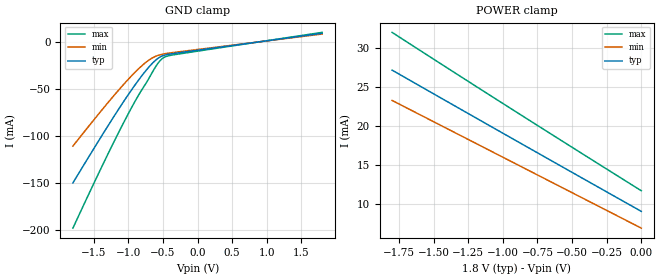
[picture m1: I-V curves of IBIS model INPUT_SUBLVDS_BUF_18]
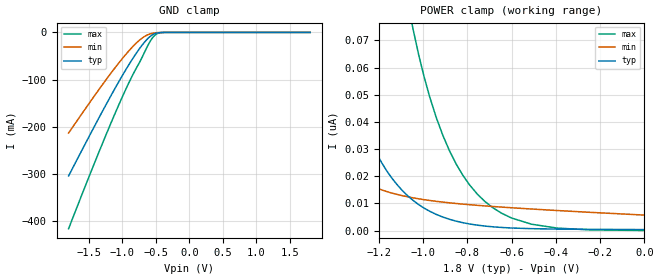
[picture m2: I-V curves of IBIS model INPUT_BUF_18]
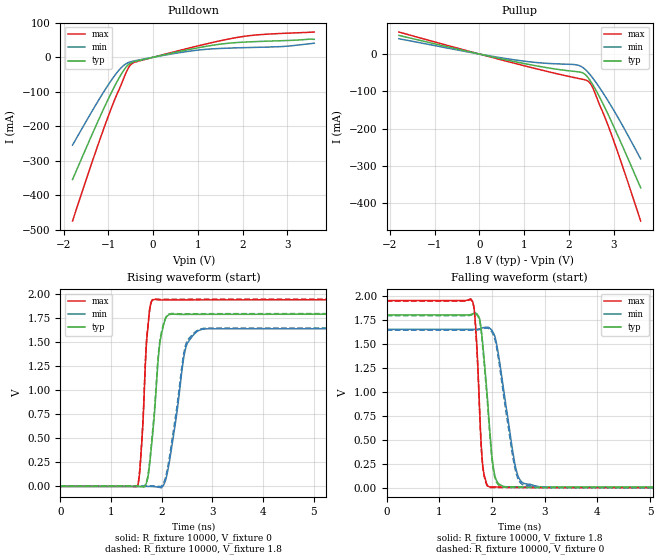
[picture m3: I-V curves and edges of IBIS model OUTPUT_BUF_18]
| TEXAS INSTRUMENTS INCORPORATED
| DLP Products
| IBIS Model of D1019WT7SV
| DLP4710 DMD
| This device can be powered at the following Vccs:
|  1.8 volt Vcc
| This file provides unique models under the [Model Selector] for each Vcc.
| For operation at a specific Vcc, select the appropriate model after each
| [Model Selector] keyword.
[IBIS Ver]   3.2
[Comment char]  |_char
[File Name]   dlp4710dmd_ibis.ibs
[File Rev]   1.0 | f_die
[Date]   October 30, 2014
[Source]   Data created from TI-SPICE simulations at TI-DLP.
[Notes]   The following is an IBIS list for the DLP4710 DMD.
##notes##|
[Disclaimer] Property of Texas Instruments Incorporated.  Unauthorized
   reproduction and/or distribution is strictly prohibited.
   This product is protected under copyright law.
   Created  2014, (C) Copyright  2014, Texas Instruments
   Incorporated, All Rights Reserved
   UNLESS THERE IS A SIGNED, WRITTEN AGREEMENT TO THE
   CONTRARY, TEXAS INSTRUMENTS (TI) IS PROVIDING THE IBIS
   MODELS  AND WITHOUT ANY WARRANTY, EXPRESSED OR
   IMPLIED.  TI assumes no liability for:
   1) the accuracy of the IBIS models provided to your
   company;
   2) the proper functioning of these IBIS Models in your
   design or for any resulting applications; or
   3) infringement of patents, copyrights or intellectual
   property rights resulting from your use of these IBIS
   models.
   TI provides IBIS Models as a service to our customers.
   You and your company shall not distribute, sell or give
   these models to anyone else without prior written
   permission from TI.
   TI reserves the right to make changes to our products or
   to discontinue any semiconductor product or service
   without notice, and advises our customers to obtain the
   latest version of relevant information to verify, before
   placing orders, that the information being relied on is
   current.
   Please be aware that your receipt and use of the IBIS
   information provided shall serve as acceptance of these
   terms and conditions.  If you do not accept these terms,
   you should return or destroy the IBIS models and any
   other accompanying information immediately.
| Component DLP4710 116-pin LGA
[Component]   DLP4710
[Manufacturer]   Texas Instruments, Inc.
[Package]
|   typ   min   max
R_pkg   7.570E-01   3.164E-01   1.297E+00
L_pkg   3.607E-09   1.961E-09   5.740E-09
C_pkg   1.200E-12   7.085E-13   1.835E-12
[Pin]   signal_name   model_name   R_pin   L_pin   C_pin
A1   VSS   GND
A5   DIE_ATT1   NC
A6   DIE_ATT2   NC
A25   NO_CONNECT   NC
A26   NO_CONNECT   NC
A27   NO_CONNECT   NC
A28   NO_CONNECT   NC
A29   NO_CONNECT   NC
A30   NO_CONNECT   NC
A31   TP0   NC
B2   VOFFSET   POWER
B3   VRESET   POWER
B4   VBIAS   POWER
B5   VSS   GND
B6   DMD_DEN_ARSTZ INPUT_BUF   9.052E-01   4.275E-09   1.384E-12
B25   VSS   GND
B26   VSS   GND
B27   VBIAS   POWER
B28   VRESET   POWER
B29   VSS   GND
B30   NO_CONNECT   NC
B31   TP1   NC
C2   VDD   POWER
C3   LS_CLK   INPUT_BUF   3.164E-01   1.985E-09   7.407E-13
C4   LS_RDATA_B   OUTPUT_BUF   5.725E-01   2.958E-09   1.053E-12
C5   VSS   GND
C6   LS_RDATA_A   OUTPUT_BUF   8.364E-01   3.940E-09   1.353E-12
C25   VSS   GND
C26   VSS   GND
C27   VSS   GND
C28   VSS   GND
C29   VOFFSET   POWER
C30   NO_CONNECT   NC
C31   TP2   NC
D1   NO_CONNECT   NC
D2   VDD   POWER
D3   LS_WDATA   INPUT_BUF   3.244E-01   1.961E-09   7.085E-13
D4   VSS   GND
D5   VSS   GND
D6   VSS   GND
D25   D_BP<3>   INPUT_SUB_LVDS_BUF   1.135E+00   5.066E-09   1.510E-12
D26   D_BN<3>   INPUT_SUB_LVDS_BUF   1.137E+00   5.148E-09   1.529E-12
D27   D_BP<2>   INPUT_SUB_LVDS_BUF   6.168E-01   3.125E-09   1.071E-12
D28   D_BN<2>   INPUT_SUB_LVDS_BUF   6.204E-01   3.145E-09   1.045E-12
D29   VDD   POWER
E1   NO_CONNECT   NC
E2   VDD   POWER
E3   D_AN<2>   INPUT_SUB_LVDS_BUF   5.618E-01   2.859E-09   9.923E-13
E4   D_AP<2>   INPUT_SUB_LVDS_BUF   5.432E-01   2.878E-09   9.777E-13
E5   D_AP<3>   INPUT_SUB_LVDS_BUF   9.821E-01   4.385E-09   1.507E-12
E6   D_AN<3>   INPUT_SUB_LVDS_BUF   9.955E-01   4.551E-09   1.508E-12
E25   VSS   GND
E26   D_BN<1>   INPUT_SUB_LVDS_BUF   9.298E-01   4.334E-09   1.370E-12
E27   D_BP<1>   INPUT_SUB_LVDS_BUF   9.101E-01   3.974E-09   1.345E-12
E28   VDDI   POWER
E29   VDD   POWER
F2   VDDI   POWER
F3   VDDI   POWER
F4   D_AN<1>   INPUT_SUB_LVDS_BUF   4.790E-01   2.676E-09   9.901E-13
F5   VSS   GND
F6   VSS   GND
F25   VSS   GND
F26   VSS   GND
F27   D_BP<0>   INPUT_SUB_LVDS_BUF   5.442E-01   2.817E-09   9.537E-13
F28   VDDI   POWER
F29   VDDI   POWER
G2   VDDI   POWER
G3   D_AN<0>   INPUT_SUB_LVDS_BUF   1.027E+00   4.332E-09   1.423E-12
G4   D_AP<1>   INPUT_SUB_LVDS_BUF   4.614E-01   2.351E-09   8.157E-13
G5   D_AN<6>   INPUT_SUB_LVDS_BUF   1.297E+00   5.740E-09   1.835E-12
G6   D_AP<6>   INPUT_SUB_LVDS_BUF   1.283E+00   5.541E-09   1.733E-12
G25   VSS   GND
G26   VSS   GND
G27   D_BN<0>   INPUT_SUB_LVDS_BUF   5.760E-01   3.075E-09   9.513E-13
G28   VDDI   POWER
G29   VDDI   POWER
H2   VDD   POWER
H3   D_AP<0>   INPUT_SUB_LVDS_BUF   1.047E+00   4.597E-09   1.623E-12
H4   VSS   GND
H5   VSS   GND
H6   VSS   GND
H25   VSS   GND
H26   DCLK_BN   INPUT_SUB_LVDS_BUF   6.634E-01   3.326E-09   1.120E-12
H27   DCLK_BP   INPUT_SUB_LVDS_BUF   6.463E-01   3.083E-09   1.177E-12
H28   VDD   POWER
H29   VDD   POWER
J2   VDD   POWER
J3   DCLK_AN   INPUT_SUB_LVDS_BUF   8.114E-01   3.591E-09   1.173E-12
J4   VSS   GND
J5   D_AN<4>   INPUT_SUB_LVDS_BUF   7.054E-01   3.488E-09   1.117E-12
J6   D_AP<4>   INPUT_SUB_LVDS_BUF   6.938E-01   3.425E-09   1.206E-12
J25   D_BP<5>   INPUT_SUB_LVDS_BUF   8.628E-01   3.997E-09   1.353E-12
J26   VSS   GND
J27   D_BP<7>   INPUT_SUB_LVDS_BUF   6.051E-01   2.936E-09   9.798E-13
J28   VDD   POWER
J29   VDD   POWER
K2   VDD   POWER
K3   DCLK_AP   INPUT_SUB_LVDS_BUF   7.998E-01   3.838E-09   1.220E-12
K4   VSS   GND
K5   VSS   GND
K6   VSS   GND
K25   D_BN<5>   INPUT_SUB_LVDS_BUF   8.634E-01   4.032E-09   1.236E-12
K26   VSS   GND
K27   D_BN<7>   INPUT_SUB_LVDS_BUF   6.261E-01   3.135E-09   1.064E-12
K28   D_BP<6>   INPUT_SUB_LVDS_BUF   5.437E-01   2.680E-09   8.685E-13
K29   VDD   POWER
L2   VDD   POWER
L3   D_AN<7>   INPUT_SUB_LVDS_BUF   4.425E-01   2.433E-09   8.918E-13
L4   D_AP<7>   INPUT_SUB_LVDS_BUF   4.361E-01   2.534E-09   8.633E-13
L5   D_AN<5>   INPUT_SUB_LVDS_BUF   8.243E-01   3.853E-09   1.367E-12
L6   D_AP<5>   INPUT_SUB_LVDS_BUF   8.277E-01   3.953E-09   1.335E-12
L25   D_BN<4>   INPUT_SUB_LVDS_BUF   1.012E+00   4.609E-09   1.430E-12
L26   D_BP<4>   INPUT_SUB_LVDS_BUF   9.928E-01   4.281E-09   1.380E-12
L27   VSS   GND
L28   D_BN<6>   INPUT_SUB_LVDS_BUF   5.805E-01   2.989E-09   1.005E-12
L29   VDD   POWER
| NOTE:  The [Diff Pin] section is commented out because the ibischk3 program
|   currently flags it as an Error when it shouldn't
| [Diff Pin]  inv_pin   vdiff   tdelay_typ
|H3   G3   200mv   NA
|G4   F4   200mv   NA
|E4   E3   200mv   NA
|E5   E6   200mv   NA
|J6   J5   200mv   NA
|L6   L5   200mv   NA
|G6   G5   200mv   NA
|L4   L3   200mv   NA
|K3   J3   200mv   NA
|F27   G27   200mv   NA
|E27   E26   200mv   NA
|D27   D28   200mv   NA
|D25   D26   200mv   NA
|L26   L25   200mv   NA
|J25   K25   200mv   NA
|K28   L28   200mv   NA
|J27   K27   200mv   NA
|H27   H26   200mv   NA
| Model INPUT_SUB_LVDS_BUF
[Model Selector]   INPUT_SUB_LVDS_BUF
INPUT_SUBLVDS_BUF_18   1.8 volt Vcc
| Model INPUT_BUF
[Model Selector]   INPUT_BUF
INPUT_BUF_18   1.8 volt Vcc
| Model OUTPUT_BUF
[Model Selector]   OUTPUT_BUF
OUTPUT_BUF_18   1.8 volt Vcc
| Models and submodels in the file (3): INPUT_SUBLVDS_BUF_18 (Input), INPUT_BUF_18 (Input), OUTPUT_BUF_18 (Output)
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[Model]   INPUT_SUBLVDS_BUF_18
Model_type  Input
Vinl=0.80
Vinh=1.00
| variable   typ   min   max
C_comp   0.69pF   0.66pF   0.72pF
[Temperature Range]   25   85   -40
[Voltage range]   1.8   1.65   1.95
[GND Clamp]
| INPUT_SUBLVDS_BUF_18
|   Voltage   I(typ)   I(min)   I(max)
-1.8V     -149.7mA   -110.7mA   -197.8mA
-1.29V    -88.84mA   -64.29mA   -118.6mA
-1.095V   -66.55mA   -47.56mA   -89.83mA
-930mV    -48.67mA   -34.42mA   -66.87mA
-790mV    -34.7mA    -24.56mA   -49.3mA
-680mV    -25.03mA   -18.39mA   -35.98mA
-580mV    -18.08mA   -14.73mA   -23.73mA
-510mV    -15.09mA   -13.26mA   -17.94mA
-450mV    -13.75mA   -12.43mA   -15.53mA
-355mV    -12.57mA   -11.45mA   -13.96mA
1.8V      8.993mA    8.203mA    9.976mA
[POWER Clamp]
| INPUT_SUBLVDS_BUF_18
|   Voltage   I(typ)   I(min)   I(max)
-1.8V     27.16mA    23.26mA    32.02mA
-1.37V    22.79mA    19.34mA    27.08mA
-920mV    18.24mA    15.23mA    21.97mA
-16.28fV  8.993mA    6.835mA    11.65mA
[Model]   INPUT_BUF_18
Model_type  Input
Vinl=0.54
Vinh=1.26
| variable   typ   min   max
C_comp   0.51pF   0.44pF   0.58pF
[Temperature Range]   25   85   -40
[Voltage range]   1.8   1.65   1.95
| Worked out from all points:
|   GND clamp passes 1 mA (typ) near -0.47 V on its own axis
[GND Clamp]
| INPUT_BUF_18
|   Voltage   I(typ)   I(min)   I(max)
-1.8V     -304mA     -213.1mA   -415.8mA
-1.52V    -227.4mA   -155.6mA   -314.4mA
-1.29V    -165.7mA   -109.6mA   -233.4mA
-1.095V   -115.3mA   -72.59mA   -167.6mA
-930mV    -75.06mA   -43.75mA   -115.2mA
-790mV    -43.93mA   -22.51mA   -75.55mA
-680mV    -22.72mA   -9.755mA   -45.56mA
-580mV    -7.998mA   -2.996mA   -17.96mA
-510mV    -2.379mA   -972.8uA   -5.564mA
-450mV    -592.5uA   -304.6uA   -1.296mA
-355mV    -35.15uA   -32.8uA    -61.22uA
1.8V      384pA      6.33nA     42.47pA
[POWER Clamp]
| INPUT_BUF_18
|   Voltage   I(typ)   I(min)   I(max)
-1.8V     438.6nA    109.4nA    1.836uA
-1.7V     293.4nA    73.99nA    1.296uA
-1.565V   164.4nA    44.27nA    784.1nA
-1.4V     75.97nA    25.31nA    401.7nA
-1.255V   36.21nA    17.25nA    210.8nA
-1.155V   20.97nA    14.17nA    130.5nA
-1.045V   11.14nA    12.07nA    74.21nA
-970mV    7.14nA     11.1nA     49.29nA
-880mV    4.163nA    10.23nA    29.33nA
-685mV    1.408nA    8.888nA    8.453nA
-395mV    567.5pA    7.406nA    949.3pA
-16.28fV  384pA      5.724nA    60.79pA
[Model]   OUTPUT_BUF_18
Model_type  Output
Vref =   0
Rref =   10000
Cref =   10p
Vmeas =   1.2
| variable   typ   min   max
C_comp   0.65pF   0.45pF   1.15pF
| C_pullup   0.66pF   0.45pF   1.15pF
| C_pulldown   0.63pF   0.50pF   1.03pF
[Temperature Range]   25   85   -40
[Voltage range]   1.8   1.65   1.95
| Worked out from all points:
|   slope of the pulldown table from 0 to 0.27 V, typ, clamps not added: 34.3 ohm
|   slope of the pullup table from 0 to 0.27 V, typ, clamps not added: 37.6 ohm
|   rising waveform, R_fixture 10000, V_fixture 0: 20-80 % time 164ps typ, 253ps min, 111ps max; typ from 0 V to 1.79 V
|   falling waveform, R_fixture 10000, V_fixture 1.8: 20-80 % time 159ps typ, 266ps min, 98.4ps max; typ from 1.8 V to 0.006 V
|   rising waveform, R_fixture 10000, V_fixture 1.8: 20-80 % time 164ps typ, 256ps min, 110ps max; typ from 0.006 V to 1.8 V
|   falling waveform, R_fixture 10000, V_fixture 0: 20-80 % time 159ps typ, 263ps min, 98.5ps max; typ from 1.79 V to 0 V
[Pulldown]
| OUTPUT_BUF_18
|   Voltage   I(typ)   I(min)   I(max)
-1.8V     -354.2mA   -254.4mA   -474.4mA
-1.265V   -195mA     -134.5mA   -266.6mA
-895mV    -92.67mA   -59.47mA   -134.6mA
-755mV    -58.61mA   -36.11mA   -91.94mA
-645mV    -35.65mA   -22.4mA    -56.96mA
-555mV    -21.67mA   -15.53mA   -31.37mA
-480mV    -15.3mA    -12.24mA   -19.11mA
-345mV    -10.18mA   -8.457mA   -11.8mA
875mV     24.33mA    18.74mA    29.04mA
1.865V    42.67mA    27.28mA    57.21mA
2.905V    48.22mA    31.33mA    69.32mA
3.6V      52.02mA    40.86mA    73.18mA
[Pullup]
| OUTPUT_BUF_18
|   Voltage   I(typ)   I(min)   I(max)
-1.8V     49.99mA    41.08mA    59.07mA
730mV     -18.9mA    -14.55mA   -23.06mA
1.36V     -33.47mA   -23.55mA   -42.08mA
2.165V    -46.93mA   -28.87mA   -64.13mA
2.32V     -51.32mA   -37.02mA   -67.96mA
2.435V    -64.68mA   -50.22mA   -73.6mA
2.49V     -74.19mA   -58.09mA   -81.45mA
2.545V    -84.87mA   -66.63mA   -94.28mA
2.7V      -119.1mA   -93.19mA   -140.9mA
2.895V    -167.2mA   -129.8mA   -198.5mA
3.195V    -246.7mA   -191.5mA   -300.4mA
3.6V      -358.2mA   -280.8mA   -447.3mA
[Ramp]
| OUTPUT_BUF_18
| variable   typ   min   max
dV/dt_r   1.08/1.67E-10   0.99/2.58E-10   1.17/1.11E-10
dV/dt_f   1.09/1.62E-10   1.00/2.72E-10   1.18/1.01E-10
R_load = 10000
[Rising Waveform]
| OUTPUT_BUF_18
R_fixture =   10000
C_fixture =   0
L_fixture =   0
V_fixture =   0
V_fixture_min = 0
V_fixture_max = 0
|   Time   V(typ)   V(min)   V(max)
0s        2.935nV    32.33nV    304.2pV
1.525ns   12.81uV    20.21uV    4.084mV
1.615ns   -3.833mV   105uV      533.5mV
1.71ns    58.13mV    123.1uV    1.568V
1.855ns   750.8mV    -2.782mV   1.947V
1.955ns   1.458V     -9.919mV   1.942V
2.08ns    1.753V     73.73mV    1.941V
2.47ns    1.791V     1.436V     1.942V
2.825ns   1.792V     1.638V     1.943V
24.99ns   1.793V     1.642V     1.944V
[Falling Waveform]
| OUTPUT_BUF_18
R_fixture =   10000
C_fixture =   0
L_fixture =   0
V_fixture =   1.8
V_fixture_min = 1.65
V_fixture_max = 1.95
|   Time   V(typ)   V(min)   V(max)
0s        1.8V       1.65V      1.95V
1.62ns    1.81V      1.65V      1.949V
1.69ns    1.819V     1.651V     1.653V
1.76ns    1.764V     1.656V     844.3mV
1.82ns    1.507V     1.667V     244.5mV
1.955ns   601.1mV    1.662V     9.6mV
2.08ns    79.45mV    1.512V     9.328mV
2.475ns   9.39mV     152mV      8.293mV
2.885ns   8.404mV    13.17mV    7.567mV
24.99ns   6.04mV     6.675mV    5.66mV
[Rising Waveform]
| OUTPUT_BUF_18
R_fixture =   10000
C_fixture =   0
L_fixture =   0
V_fixture =   1.8
V_fixture_min = 1.65
V_fixture_max = 1.95
|   Time   V(typ)   V(min)   V(max)
0s        6.039mV    6.675mV    5.66mV
1.525ns   6.058mV    6.695mV    10.55mV
1.61ns    2.738mV    6.771mV    514.5mV
1.71ns    72.65mV    6.795mV    1.588V
1.855ns   789.8mV    4.171mV    1.952V
1.955ns   1.486V     187.2uV    1.948V
2.08ns    1.761V     104.7mV    1.948V
2.465ns   1.798V     1.459V     1.948V
2.825ns   1.798V     1.646V     1.949V
24.99ns   1.8V       1.65V      1.95V
[Falling Waveform]
| OUTPUT_BUF_18
R_fixture =   10000
C_fixture =   0
L_fixture =   0
V_fixture =   0
V_fixture_min = 0
V_fixture_max = 0
|   Time   V(typ)   V(min)   V(max)
0s        1.793V     1.642V     1.944V
1.62ns    1.803V     1.642V     1.942V
1.69ns    1.811V     1.643V     1.63V
1.76ns    1.748V     1.648V     814.7mV
1.815ns   1.504V     1.657V     253.2mV
1.955ns   560.3mV    1.649V     4.112mV
2.075ns   66.14mV    1.49V      3.651mV
2.465ns   3.348mV    135.5mV    2.653mV
2.86ns    2.404mV    7.718mV    1.943mV
24.99ns   6.498nV    37.43nV    3.212nV
